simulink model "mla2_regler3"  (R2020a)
settings: Solver=ode5  StartTime=0.0  StopTime=7  FixedStep=0.0001  RelTol=1e-4  EnableMultiTasking=on
PreLoadFcn:
  | MLA_Sensor1 = load('mla_sensor1.dat');
libraries: libmla x1, simulink_need_slupdate x1

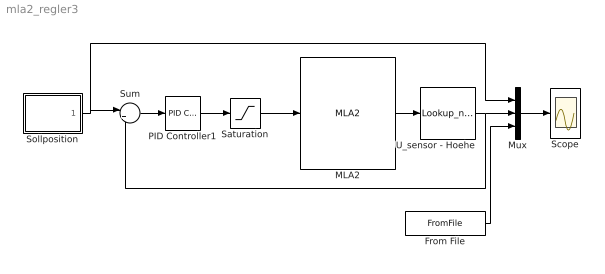
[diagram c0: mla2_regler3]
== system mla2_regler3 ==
  From File : FromFile  FileName=mla_regler3.mat  SampleTime=0
  MLA2 : libmla/MLA2  g=9.81  m=0.125  Fr_g=0.14  Fr_h=0.1  d_l=0.18  d_t=0.1  a=40691  b=0.0687  N=4.282
  Mux : Mux  Inputs=3
  PID Controller1 : simulink_need_slupdate/PID Controller  P=9000  I=2000  D=100
  Saturation : Saturate  UpperLimit=3  LowerLimit=-3
  Scope : Scope
  Sollposition : Subsystem
  Sum : Sum  Inputs=|+-
  U_sensor - Hoehe : Lookup_n-D  NumberOfTableDimensions=1  BreakpointsForDimension1=MLA_Sensor1(:,1)  Table=MLA_Sensor1(:,2)  RndMeth=Simplest
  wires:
  MLA2/1 -> U_sensor - Hoehe/1
  Mux/1 -> Scope/1
  Sum/1 -> PID Controller1/1
  Sollposition/1(Sollwert) -> Sum/1, Mux/1
  U_sensor - Hoehe/1 -> Mux/2, Sum/2
  PID Controller1/1 -> Saturation/1
  Saturation/1 -> MLA2/1
  From File/1 -> Mux/3

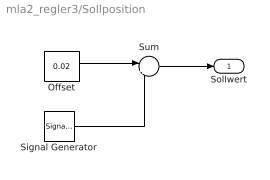
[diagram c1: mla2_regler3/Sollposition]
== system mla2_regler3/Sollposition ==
  Offset : Constant  Value=0.02
  Signal Generator : SignalGenerator  Amplitude=0.01  Frequency=0.5
  Sum : Sum  Inputs=|++
  Sollwert : Outport
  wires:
  Offset/1 -> Sum/1
  Sum/1 -> Sollwert/1
  Signal Generator/1 -> Sum/2
